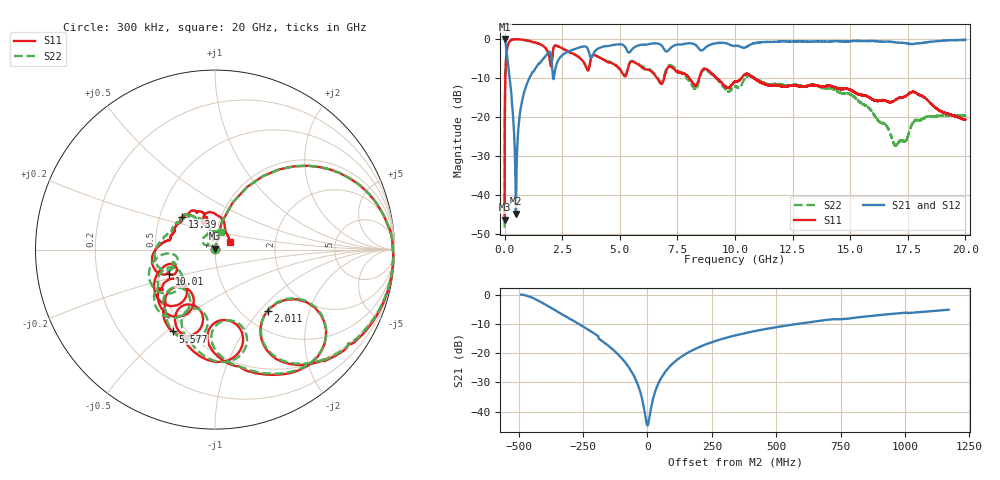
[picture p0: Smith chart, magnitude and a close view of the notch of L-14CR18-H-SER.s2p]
!{L-14CR18}
!Johanson Technology Inc.
!www.johansontechnology.com
!Test Board Conditions:
!Substrate Type  RO4350B
!Substrate Thickness  20 mil
!Substrate Dk  3.66
!TL Type: GCPW
!TL Trace Width  36 mil
!TL Gap  12 mil
!Electrode orientation  Horizontal
!DUT TOPOLOGY	SERIES
!Mounting Pad LxW  26x36 mil
! Created Sun Jun 20 13:11:47 2021
# hz S ma R 50
! 2 Port Network Data from SP1.SP block
! freq  magS11  angS11  magS21  angS21  magS12  angS12  magS22  angS22
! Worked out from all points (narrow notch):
!   20001 points, 300 kHz to 20 GHz, reference 50 ohm
!   highest |S21| = 0.00 dB at 300 kHz (marker M1); lowest = -44.7 dB at 490.3 MHz (marker M2)
!   notch at M2: 43.6 dB deep, 195 MHz wide at half that depth
!   lowest |S11| = -46.2 dB at 300 kHz (marker M3), VSWR 1.01, Z = 50 + j0.486 ohm
!   |S11| at or under -10 dB: 8.011 GHz to 8.445 GHz (433.9 MHz wide, 5.27 % of centre); 9.21 GHz to 10.28 GHz (1.071 GHz wide, 11 % of centre); 10.82 GHz to end of sweep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
!   |S22| runs from -48.3 to 0.0 dB; largest |S21 - S12| = 0.011
!   S11 on the Smith chart (normalised r, x): 300 kHz: 1.00, +0.01; 2.011 GHz: 1.30, -1.11; 5.577 GHz: 0.42, -0.53; 10.01 GHz: 0.58, -0.17; 13.39 GHz: 0.65, +0.26; 20 GHz: 1.18, +0.09
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300000  0.004882 84.2  0.9998 -0.2  0.9967 -0.3  0.003858 77.0
1.233e8  0.7984 33.2  0.5667 -54.3  0.5677 -54.3  0.7995 33.2
4.903e8  0.9938 -5.1  0.005817 -3.5  0.005765 -3.6  0.993 -5.0
6.973e8  0.9882 -14.6  0.13 73.3  0.1301 73.4  0.9847 -14.5
9.413e8  0.9663 -24.4  0.2537 65.2  0.254 65.1  0.9624 -24.4
1.7073e9  0.8038 -53.0  0.571 35.3  0.5728 35.3  0.7998 -52.6
2.0113e9  0.4491 -49.1  0.635 -2.8  0.6359 -2.7  0.4468 -48.4
2.1613e9  0.8163 -43.0  0.3544 25.8  0.3547 25.9  0.8128 -42.5
2.3893e9  0.7913 -61.4  0.5718 25.6  0.5718 25.6  0.7869 -60.9
3.3343e9  0.5511 -92.4  0.7957 -5.6  0.7958 -5.6  0.549 -90.4
5.5773e9  0.5134 -117.3  0.7614 -36.7  0.7609 -36.7  0.5225 -113.8
6.6673e9  0.3011 -136.4  0.8739 -62.1  0.8755 -62.0  0.3105 -137.2
7.1943e9  0.4448 -130.5  0.7628 -59.2  0.7632 -59.1  0.4648 -132.6
8.2493e9  0.2572 -137.7  0.8545 -83.7  0.8557 -83.6  0.2319 -150.0
1.00003e10  0.2861 -151.4  0.819 -102.8  0.8183 -102.7  0.2481 -162.2
1.00103e10  0.2873 -151.9  0.8176 -102.9  0.8206 -102.8  0.2474 -162.3
1.33343e10  0.2588 135.7  0.9274 -142.5  0.9249 -142.4  0.2592 133.7
1.33893e10  0.2588 134.6  0.9294 -142.9  0.9254 -143.1  0.2595 132.3
1.66673e10  0.157 111.8  0.929 171.9  0.9288 172.3  0.06947 101.3
1.69943e10  0.1691 115.9  0.9065 167.2  0.9073 167.4  0.0436 126.0
1.78293e10  0.2062 93.5  0.8727 160.6  0.876 160.5  0.09098 135.5
2e10  0.09219 25.1  0.974 131.9  0.9736 131.9  0.1042 71.6
